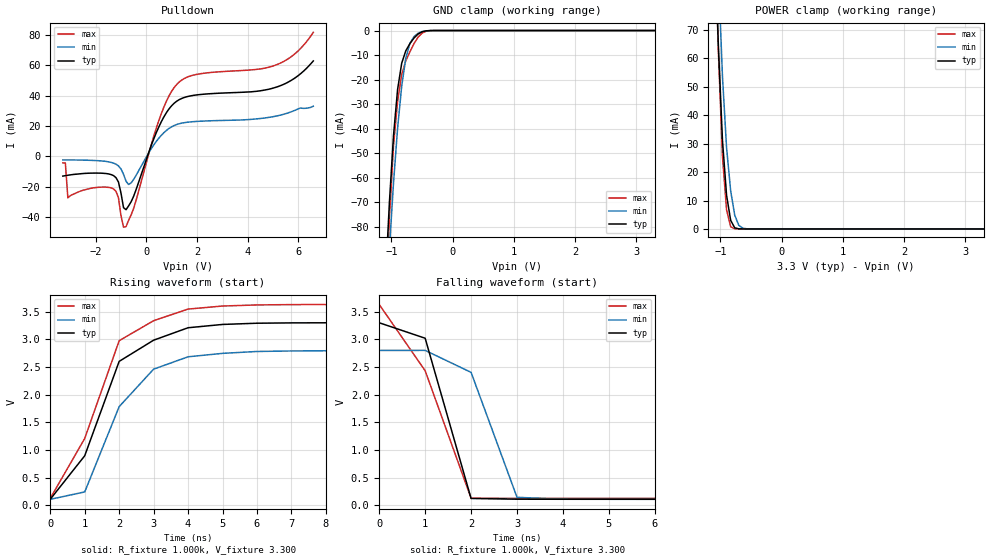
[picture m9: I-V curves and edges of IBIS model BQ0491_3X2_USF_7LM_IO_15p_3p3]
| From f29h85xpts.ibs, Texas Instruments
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|   Model BQ0491_3X2_USF_7LM_IO_15p_3p3
[Model]   BQ0491_3X2_USF_7LM_IO_15p_3p3
Model_type   I/O_open_drain
Polarity   Non-Inverting
Enable   Active-Low
Vinl =   0.800V
Vinh =   2.000V
Vmeas =  1.650V
Cref =   15.000pF
Rref =   1.000k
Vref =   3.300V
|   typ   min   max
C_comp   1.084pF   1.003pF   1.123pF
[Model Spec]
Vinh   2.000V   2.000V   2.000V
Vinl   0.800V   0.800V   0.800V
[Temperature Range]   25   155   -40
[Voltage Range]   3.300V   2.800V   3.630V
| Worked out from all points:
|   slope of the pulldown table from 0 to 0.495 V, typ, clamps not added: 22.9 ohm
|   GND clamp passes 1 mA (typ) near -0.53 V on its own axis
|   POWER clamp passes 1 mA (typ) near -0.78 V on its own axis
|   rising waveform, R_fixture 1.000k, V_fixture 3.300: 20-80 % time 1.34ns typ, 1.44ns min, 1.33ns max; typ from 0.11 V to 3.3 V
|   falling waveform, R_fixture 1.000k, V_fixture 3.300: 20-80 % time 661ps typ, 715ps min, 1.11ns max; typ from 3.3 V to 0.109 V
[Pulldown]
|Voltage   I(typ)   I(min)   I(max)
-3.3V     -13.02mA   -2.341mA   -4.302mA
-3.2V     -12.73mA   -2.339mA   -4.378mA
-3.1V     -12.44mA   -2.348mA   -27.4mA
-1.3V     -12.63mA   -4.385mA   -21.46mA
-1.1V     -16.94mA   -6.32mA    -27.31mA
-900mV    -33.86mA   -11.82mA   -46.69mA
-800mV    -35.16mA   -16.44mA   -46.35mA
-600mV    -29.91mA   -17.47mA   -38.61mA
500mV     19.63mA    12.11mA    23.89mA
1.2V      36.37mA    21mA       47.41mA
5.1V      45.45mA    26.47mA    60.14mA
6.6V      62.95mA    33.05mA    81.82mA
[GND_clamp]
|Voltage   I(typ)   I(min)   I(max)
-3.3V     -1.477A    -1.275A    -1.767A
-1.1V     -102.3mA   -117.4mA   -113.6mA
-1.033V   -69.65mA   -88.47mA   -75.69mA
-967mV    -42.74mA   -62.14mA   -47.03mA
-900mV    -23.95mA   -39.73mA   -28.88mA
-833mV    -13.31mA   -22.62mA   -17.87mA
-767mV    -8.284mA   -11.35mA   -12.33mA
-700mV    -5.36mA    -5.295mA   -8.734mA
-567mV    -1.453mA   -1.127mA   -2.734mA
-433mV    -123uA     -137uA     -288.6uA
-300mV    -2.171uA   -7.759uA   -7.425uA
3.3V      0A         0A         0A
[POWER_clamp]
|Voltage   I(typ)   I(min)   I(max)
-3.3V     1.901A     2.191A     2.069A
-1.1V     105.6mA    134.8mA    109.4mA
-1.033V   63.91mA    89.93mA    62.06mA
-967mV    31.18mA    53.67mA    25.42mA
-900mV    11.84mA    28.57mA    6.708mA
-833mV    3.029mA    13.38mA    772.2uA
-767mV    401uA      4.887mA    44.81uA
-700mV    39.91uA    1.256mA    4.584uA
-633mV    5.004uA    258.3uA    1.413uA
-567mV    1.057uA    50.08uA    519.1nA
3.3V      0A         0A         0A
[Ramp]
| variable   typ   min   max
dV/dt_r   1.914/1.296n   1.615/1.263n   2.103/1.336n
dV/dt_f   1.914/0.125n   1.615/0.208n   2.103/98.310p
R_load = 1.000k
[Rising Waveform]
R_fixture= 1.000k
V_fixture= 3.300
V_fixture_min= 2.800
V_fixture_max= 3.630
|time   V(typ)   V(min)   V(max)
0s        110.1mV    108.6mV    126.7mV
1ns       896.2mV    242.3mV    1.208V
2ns       2.602V     1.784V     2.976V
3ns       2.985V     2.462V     3.337V
4ns       3.21V      2.685V     3.547V
5ns       3.27V      2.747V     3.602V
6ns       3.292V     2.781V     3.622V
9ns       3.3V       2.796V     3.63V
50us      3.3V       2.8V       3.63V
[Falling Waveform]
R_fixture= 1.000k
V_fixture= 3.300
V_fixture_min= 2.800
V_fixture_max= 3.630
|time   V(typ)   V(min)   V(max)
0s        3.299V     2.8V       3.63V
1ns       3.02V      2.8V       2.432V
2ns       123.8mV    2.403V     128.2mV
3ns       110.5mV    144.6mV    125.7mV
4ns       109.4mV    109.8mV    125.7mV
21ns      109.3mV    108.1mV    125.7mV
50us      109.3mV    108.1mV    125.7mV
